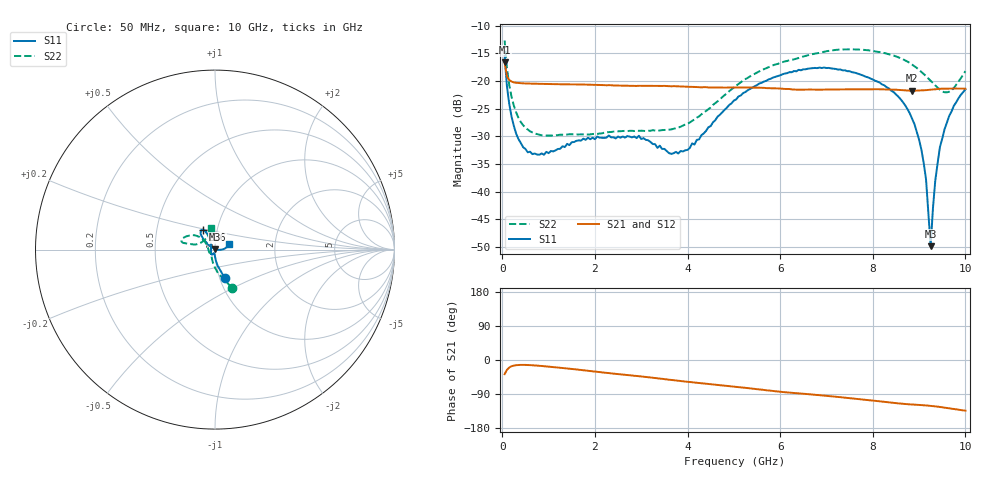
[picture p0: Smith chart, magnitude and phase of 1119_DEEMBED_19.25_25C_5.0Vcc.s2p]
!Hittite Microwave Corp.
!Digital Attenuator/PhaseShifter Rev 1.4.0
!Filename: C:\DATA\DATA\1119_DEEMBED_19.25_25C_5.0Vcc.s2p
!VNA ID: Agilent Technologies,N5224A,MY51441122,A.10.45.03
!Device type:
!2 Port Calibration.
!Temp(C): 25
!Lot Number:
!Serial Number:
!Operator:
!Misc:
!Attenuator:  19.250
# GHZ S DB R 50.0
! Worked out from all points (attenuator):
!   200 points, 50 MHz to 10 GHz, reference 50 ohm
!   highest |S21| = -16.65 dB at 50 MHz (marker M1); lowest = -21.8 dB at 8.85 GHz (marker M2)
!   lowest |S11| = -49.8 dB at 9.25 GHz (marker M3), VSWR 1.01, Z = 50.1 + j0.311 ohm
!   |S11| at or under -10 dB: start of sweep to end of sweep
!   |S22| runs from -29.9 to -12.7 dB; largest |S21 - S12| = 0.00023
!   S11 on the Smith chart (normalised r, x): 50 MHz: 1.06, -0.35; 6.6 GHz: 0.85, +0.19; 10 GHz: 1.17, +0.07
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0.05  -15.47 -71.0  -16.65 -37.4  -16.65 -37.4  -12.67 -65.9
0.1  -20.93 -81.0  -19.15 -26.0  -19.14 -26.0  -17.61 -83.1
0.2  -26.45 -87.9  -20.10 -16.5  -20.10 -16.5  -22.88 -99.8
0.35  -30.50 -92.4  -20.36 -13.1  -20.37 -13.1  -26.67 -113.8
0.55  -32.88 -98.5  -20.45 -13.2  -20.45 -13.2  -28.77 -125.3
1.75  -30.42 -121.3  -20.63 -27.0  -20.63 -27.1  -29.64 -138.9
2.95  -29.89 -131.6  -20.86 -42.7  -20.87 -42.7  -29.00 -157.9
3.4  -31.68 -153.2  -20.89 -49.0  -20.89 -49.0  -28.93 -171.2
4  -32.45 153.0  -21.04 -57.4  -21.05 -57.5  -27.75 164.6
5.05  -23.33 116.2  -21.17 -70.7  -21.19 -70.7  -20.85 140.0
6.6  -17.77 121.9  -21.55 -90.1  -21.56 -90.1  -15.35 153.8
6.7  -17.70 122.8  -21.54 -91.3  -21.55 -91.3  -15.13 154.8
7.5  -18.23 131.2  -21.51 -100.7  -21.52 -100.8  -14.26 164.0
8.35  -21.34 137.8  -21.53 -111.8  -21.53 -111.7  -15.15 167.9
8.85  -26.83 142.4  -21.75 -117.4  -21.75 -117.4  -17.04 167.5
9.1  -34.82 143.8  -21.68 -119.5  -21.69 -119.5  -18.73 165.7
9.15  -37.75 143.5  -21.65 -119.9  -21.66 -119.9  -19.12 164.8
9.25  -49.84 74.3  -21.56 -121.0  -21.58 -121.1  -19.96 161.7
9.35  -37.96 -0.9  -21.49 -122.4  -21.50 -122.4  -20.79 156.7
9.45  -31.93 -4.1  -21.40 -124.0  -21.41 -124.0  -21.59 149.1
9.65  -26.31 3.6  -21.37 -127.5  -21.38 -127.4  -21.93 127.2
10  -21.53 20.3  -21.40 -133.7  -21.40 -133.7  -18.22 99.7
